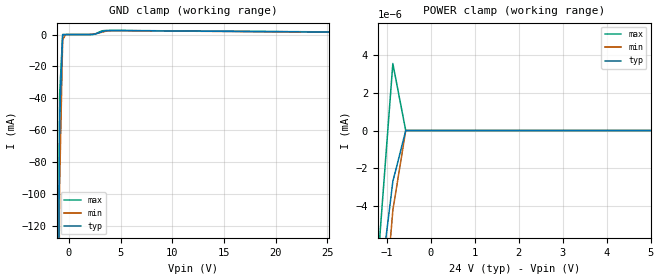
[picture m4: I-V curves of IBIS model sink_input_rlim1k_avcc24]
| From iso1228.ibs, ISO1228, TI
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|   Model sink_input_rlim1k_avcc24
[Model] sink_input_rlim1k_avcc24
Model_type Input
Vinl =  5.100V
Vinh =  6.000V
C_comp   0.859pF   0.874pF   1.06pF
[Model Spec]
Vinh   6.000V   5.700V   6.400V
Vinl   5.100V   4.700V   5.300V
[Temperature Range]   27.000   150   -40
[Voltage Range]   24.000V   24.000V   24.000V
[GND_clamp]
|Voltage   I(typ)   I(min)   I(max)
-24V      -39.17A    -38.93A    -39.33A
-1.192V   -364.9mA   -400.1mA   -356.7mA
-899mV    -54.96mA   -94.69mA   -37.61mA
-606mV    -31.63uA   -3.096mA   -1.266uA
-313mV    -342.2nA   -2.087uA   -415.5nA
2.323V    104.3uA    260.2uA    82.14uA
3.202V    1.817mA    1.503mA    2.359mA
4.374V    2.522mA    2.433mA    2.596mA
48V       517.9uA    330.2uA    691.7uA
[POWER_clamp]
|Voltage   I(typ)   I(min)   I(max)
-24V      1.792A     2.02A      3.929A
-11.4V    5.613uA    128.4nA    54.43uA
-11.11V   5.282uA    -110.5nA   44.64uA
-7.01V    157.5nA    -1.111uA   4.347uA
-6.717V   -225.8nA   -1.01uA    3.839uA
-4.667V   -315nA     -445.9nA   246.2nA
-4.374V   -271.8nA   -385nA     -190.8nA
-1.152V   -8.282nA   -12.41nA   -5.512nA
-859mV    -2.701nA   -4.225nA   3.545nA
-566mV    0A         0A         0A
5V        0A         0A         0A
